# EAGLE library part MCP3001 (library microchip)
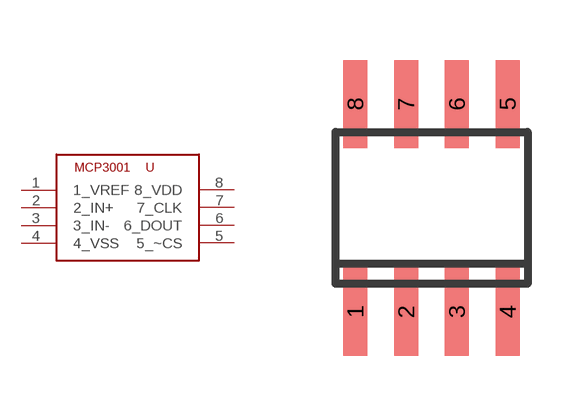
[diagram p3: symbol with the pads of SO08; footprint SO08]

Designator prefix -

## MCP3001  [SO08]
1  1_VREF
2  2_IN+
3  3_IN-
4  4_VSS
5  5_~CS
6  6_DOUT
7  7_CLK
8  8_VDD

## Footprint SO08 (pad centres in mm)
Small Outline Package
smd 0.6 x 2.2: 1 -1.905,-2.6; 2 -0.635,-2.6; 3 0.635,-2.6; 4 1.905,-2.6; 5 1.905,2.6; 6 0.635,2.6; 7 -0.635,2.6; 8 -1.905,2.6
